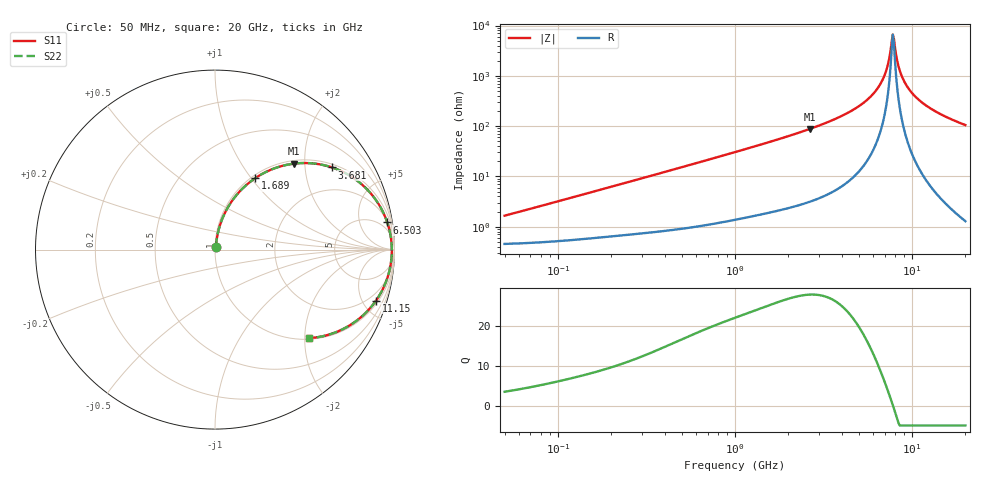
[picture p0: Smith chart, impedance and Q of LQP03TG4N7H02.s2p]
!Murata Part Number: LQP03TG4N7H02
!These Parameters are Measured in Series Mode Connection
!  o--[Z]--o
!Port1  Port2
!  o-------o
!Freq. Start=50[MHz] Stop=20[GHz], 401[Steps]
# Hz S RI R 50
!Freq.(Hz) S11(Real) S11(Imag) S21(Real) S21(Imag) S12(Real) S12(Imag) S22(Real) S22(Imag)
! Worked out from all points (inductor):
!   401 points, 50 MHz to 20 GHz, reference 50 ohm
!   read as one part in series: L = 5.06 nH near 51.52 MHz
!   highest Q = 28 at 2.647 GHz (marker M1), where L = 5.29 nH
!   self-resonance near 7.784 GHz
!   S11 on the Smith chart (normalised r, x): 50 MHz: 1.01, +0.03; 1.689 GHz: 1.04, +1.05; 3.681 GHz: 1.11, +2.77; 6.503 GHz: 2, +12; 11.15 GHz: 1.25, -6.24; 20 GHz: 1.03, -2.10
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5e7  0.00477 0.0158  0.9952 -0.0158  0.9952 -0.0158  0.00477 0.0158
1.364002e8  0.0074 0.0421  0.9926 -0.0421  0.9926 -0.0421  0.0074 0.0421
3.721004e8  0.0204 0.1104  0.9796 -0.1104  0.9796 -0.1104  0.0204 0.1104
1e9  0.0948 0.2712  0.9052 -0.2712  0.9052 -0.2712  0.0948 0.2712
1.689197e9  0.2246 0.3985  0.7754 -0.3985  0.7754 -0.3985  0.2246 0.3985
2.647493e9  0.4386 0.4787  0.5614 -0.4787  0.5614 -0.4787  0.4386 0.4787
2.728004e9  0.4566 0.4806  0.5434 -0.4806  0.5434 -0.4806  0.4566 0.4806
3.680849e9  0.6529 0.4575  0.3471 -0.4575  0.3471 -0.4575  0.6529 0.4575
5.194772e9  0.869 0.3118  0.131 -0.3118  0.131 -0.3118  0.869 0.3118
5.856089e9  0.9247 0.2313  0.0753 -0.2313  0.0753 -0.2313  0.9247 0.2313
6.503449e9  0.9599 0.1513  0.0401 -0.1513  0.0401 -0.1513  0.9599 0.1513
7.009217e9  0.9761 0.0902  0.0239 -0.0902  0.0239 -0.0902  0.9761 0.0902
7.222371e9  0.9804 0.0652  0.0196 -0.0652  0.0196 -0.0652  0.9804 0.0652
7.442007e9  0.9833 0.0399  0.0167 -0.0399  0.0167 -0.0399  0.9833 0.0399
7.668323e9  0.985 0.0145  0.015 -0.0145  0.015 -0.0145  0.985 0.0145
7.901521e9  0.9853 -0.011  0.0147 0.011  0.0147 0.011  0.9853 -0.011
8.389408e9  0.9819 -0.0618  0.0181 0.0618  0.0181 0.0618  0.9819 -0.0618
8.907419e9  0.9733 -0.112  0.0267 0.112  0.0267 0.112  0.9733 -0.112
9.745021e9  0.9508 -0.1846  0.0492 0.1846  0.0492 0.1846  0.9508 -0.1846
1.115139e10  0.8975 -0.2836  0.1025 0.2836  0.1025 0.2836  0.8975 -0.2836
1.438523e10  0.7495 -0.4227  0.2505 0.4227  0.2505 0.4227  0.7495 -0.4227
2e10  0.5235 -0.4934  0.4765 0.4934  0.4765 0.4934  0.5235 -0.4934
